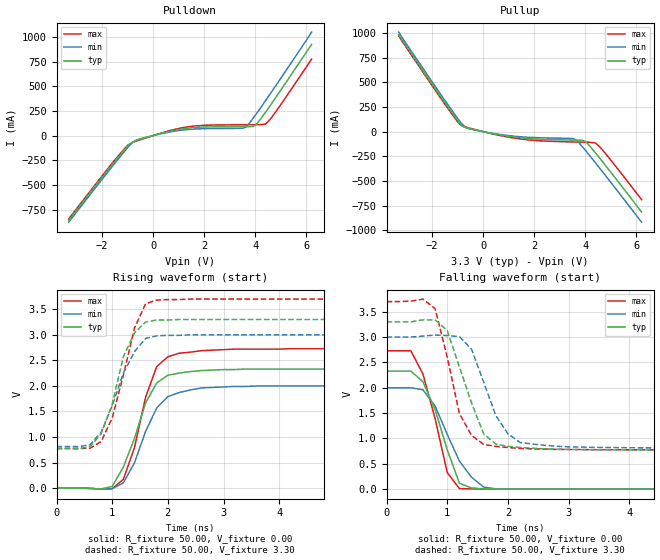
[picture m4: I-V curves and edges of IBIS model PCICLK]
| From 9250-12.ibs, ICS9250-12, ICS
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|   Model PCICLK
[Model]   PCICLK
Model_type   Output
Polarity   Non-Inverting
Vmeas = 1.5V
Cref = 30pF
Rref = 0
Vref = 1.5V
C_comp   5.50pF   5.00pF   6.00pF
[Temperature Range]   27.00   70.00   0.00
[Voltage Range]   3.30V   3.00V   3.70V
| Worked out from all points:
|   slope of the pulldown table from 0 to 0.495 V, typ, clamps not added: 14.5 ohm
|   slope of the pullup table from 0 to 0.495 V, typ, clamps not added: 18.8 ohm
|   rising waveform, R_fixture 50.00, V_fixture 0.00: 20-80 % time 480ps typ, 475ps min, 414ps max; typ from 0 V to 2.33 V
|   rising waveform, R_fixture 50.00, V_fixture 3.30: 20-80 % time 420ps typ, 487ps min, 401ps max; typ from 0.772 V to 3.3 V
|   falling waveform, R_fixture 50.00, V_fixture 0.00: 20-80 % time 401ps typ, 482ps min, 339ps max; typ from 2.33 V to 0 V
|   falling waveform, R_fixture 50.00, V_fixture 3.30: 20-80 % time 445ps typ, 450ps min, 367ps max; typ from 3.3 V to 0.772 V
[Pulldown]
| voltage   I(typ)   I(min)   I(max)
-3.3V     -857.8mA   -878.3mA   -845.1mA
-1.5V     -260.9mA   -281.8mA   -248.1mA
-1V       -106.4mA   -124.1mA   -99.56mA
-700mV    -54.41mA   -51.21mA   -59.61mA
300mV     21.43mA    18mA       24.36mA
1.3V      73.78mA    60.41mA    86.54mA
2.1V      87.67mA    70.65mA    105.3mA
3.6V      91.32mA    82.18mA    110.4mA
4V        105.2mA    207.1mA    111.2mA
4.4V      237.4mA    355.2mA    116.5mA
4.8V      387.1mA    507mA      242.1mA
6.2V      925.7mA    1.05A      776.2mA
[Pullup]
| voltage   I(typ)   I(min)   I(max)
-3.3V     983.7mA    1.01A      969.4mA
-1.5V     295.3mA    319.2mA    280.6mA
-900mV    81.81mA    102.4mA    72.29mA
-800mV    56.16mA    70.86mA    55.66mA
-600mV    36.42mA    32.43mA    40.85mA
500mV     -26.52mA   -22.39mA   -30.58mA
1.9V      -72.3mA    -58.7mA    -86.64mA
3.6V      -85.61mA   -78.64mA   -105.1mA
4V        -101.2mA   -188.8mA   -107.1mA
4.4V      -216.9mA   -317.6mA   -115.3mA
4.8V      -347.1mA   -449.6mA   -225.3mA
6.2V      -815.5mA   -918.7mA   -690mA
[Ramp]
| variable   typ   min   max
dV/dt_r   1.40/423.41p   1.20/453.67p   1.64/371.16p
dV/dt_f   1.52/300.00p   1.31/400.00p   1.75/300.00p
[Rising Waveform]
R_fixture = 50.00
V_fixture = 0.00
V_fixture_min = 0.00
V_fixture_max = 0.00
| time   V(typ)   V(min)   V(max)
0s        0V         0V         0V
1ns       32.22mV    -10.64mV   -13.29mV
1.2ns     411.2mV    102mV      172mV
1.4ns     970.3mV    494.5mV    791mV
1.6ns     1.67V      1.11V      1.78V
1.8ns     2.06V      1.57V      2.38V
2ns       2.21V      1.79V      2.57V
2.2ns     2.25V      1.87V      2.64V
3.6ns     2.33V      2V         2.72V
10ns      2.33V      2V         2.73V
[Rising Waveform]
R_fixture = 50.00
V_fixture = 3.30
V_fixture_min = 3.00
V_fixture_max = 3.70
| time   V(typ)   V(min)   V(max)
0s        772.3mV    812.8mV    776.4mV
400ps     772.1mV    812.6mV    776.3mV
600ps     808.1mV    845.3mV    778.7mV
800ps     1.06V      1.09V      909.8mV
1ns       1.64V      1.61V      1.37V
1.2ns     2.57V      2.25V      2.21V
1.4ns     3.04V      2.67V      3.13V
1.6ns     3.25V      2.93V      3.61V
1.8ns     3.29V      2.98V      3.68V
10ns      3.3V       3V         3.7V
[Falling Waveform]
R_fixture = 50.00
V_fixture = 0.00
V_fixture_min = 0.00
V_fixture_max = 0.00
| time   V(typ)   V(min)   V(max)
0s        2.33V      2V         2.73V
400ps     2.33V      2V         2.73V
600ps     2.12V      1.96V      2.27V
800ps     1.57V      1.64V      1.39V
1ns       775.6mV    1.08V      325.8mV
1.2ns     116.9mV    554.2mV    11.96mV
1.4ns     24.29mV    235.1mV    6.19mV
1.6ns     4.66mV     39.83mV    3.23mV
1.8ns     3.42mV     7.62mV     2.36mV
10ns      4.18uV     -6.16uV    896.5nV
[Falling Waveform]
R_fixture = 50.00
V_fixture = 3.30
V_fixture_min = 3.00
V_fixture_max = 3.70
| time   V(typ)   V(min)   V(max)
0s        3.3V       3V         3.7V
600ps     3.34V      3.02V      3.75V
800ps     3.34V      3.04V      3.56V
1ns       3.13V      3.03V      2.6V
1.2ns     2.41V      3.01V      1.49V
1.4ns     1.7V       2.76V      1.06V
1.6ns     1.09V      2.11V      881.7mV
2ns       844.8mV    1.09V      822.1mV
2.4ns     809mV      889.9mV    795.5mV
10ns      772.3mV    812.8mV    776.4mV
